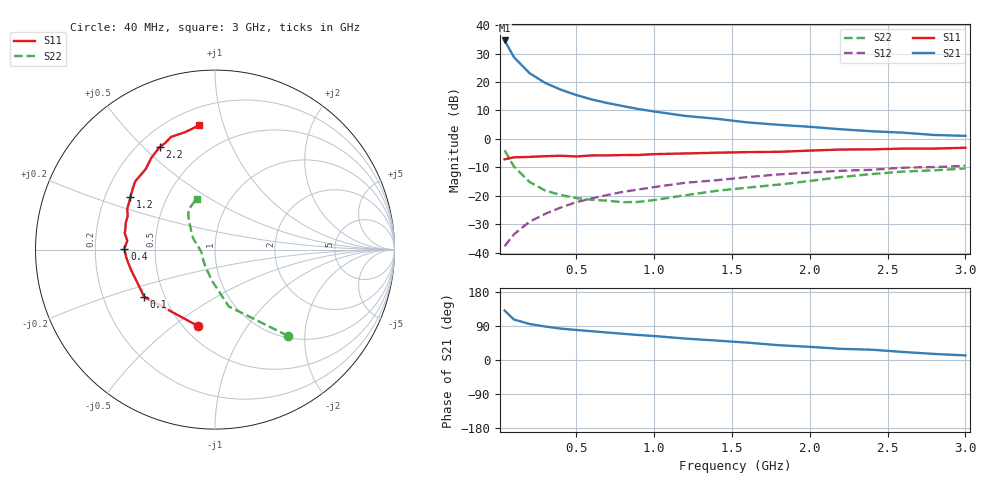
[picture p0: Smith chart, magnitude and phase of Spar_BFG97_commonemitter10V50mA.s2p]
! Filename:  BFG97G.S2P  Version:  2.0
! NXP part #: BFG97  Date: Jul 1990
! Bias condition: Vce=10V, Ic=50mA
#  MHz  S  MA  R  50
! Freq  S11  S21  S12  S22  !GUM [dB]
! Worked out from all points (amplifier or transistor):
!   21 points, 40 MHz to 3 GHz, reference 50 ohm
!   highest |S21| = 34.6 dB at 40 MHz (marker M1)
!   |S21| within 3 dB of that: start of sweep to 70.56 MHz
!   unconditionally stable (mu >= 1): 258.7 MHz to 2.994 GHz
!   at 300 MHz: K = 1.03, MAG = 22.0 dB, |S12| = -26.4 dB
!   at 1 GHz: K = 1.07, MAG = 11.6 dB, |S12| = -17.0 dB
!   at 3 GHz: K = 1.00, MSG = 5.3 dB, |S12| = -9.5 dB
!   S11 on the Smith chart (normalised r, x): 40 MHz: 0.59, -0.62; 100 MHz: 0.39, -0.26; 400 MHz: 0.33, +0.00; 1.2 GHz: 0.31, +0.26; 2.2 GHz: 0.28, +0.56; 3 GHz: 0.31, +0.83
40  0.437 -102.2  53.67 130.5  0.013 61.1  0.629 -49.8
100  0.474 -146.2  27.24 106.8  0.021 60.7  0.326 -76.3
200  0.482 -166.9  14.29 95.1  0.035 67.9  0.175 -95.5
300  0.496 -174.8  9.637 88.4  0.048 69.1  0.124 -110.5
400  0.505 179.5  7.339 82.9  0.062 69.9  0.103 -123.7
500  0.491 174.2  5.901 79.2  0.077 70.3  0.091 -133.9
600  0.511 169.7  4.931 75.9  0.09 69.9  0.085 -143.1
700  0.513 166.5  4.261 72.5  0.103 69.3  0.082 -152.8
800  0.519 163.6  3.772 69.2  0.117 67.9  0.077 -162.6
900  0.521 159.0  3.344 66.0  0.129 67.0  0.078 -172.4
1000  0.539 155.1  3.03 63.3  0.142 65.6  0.084 -179.9
1200  0.554 148.2  2.534 56.6  0.169 63.5  0.102 164.6
1400  0.571 143.4  2.259 51.3  0.187 60.3  0.122 157.5
1600  0.585 139.3  1.947 45.8  0.213 58.6  0.139 152.0
1800  0.592 130.7  1.767 39.1  0.237 53.9  0.157 145.6
2000  0.622 124.8  1.63 34.7  0.256 52.2  0.182 138.3
2200  0.649 118.4  1.474 29.5  0.275 49.4  0.213 132.7
2400  0.655 115.2  1.36 27.1  0.286 48.5  0.241 128.3
2600  0.674 111.2  1.285 21.2  0.312 44.2  0.266 123.5
2800  0.675 104.4  1.17 16.0  0.319 39.7  0.28 117.3
3000  0.698 97.2  1.13 12.1  0.335 38.1  0.302 109.8
